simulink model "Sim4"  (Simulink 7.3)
settings: Solver=ode45  StartTime=0.0  StopTime=60  FixedStep=0.01  RelTol=1e-3
InitFcn:
  | r2d=180/pi; d2r=pi/180;
  | om=1.2; zt=0.14; Kp=om^2; Kr=2*zt*om; %frq;
  | [Ad, Bd, Cd, Dd]= later_des;
  | [An, Bn, Cn, Dn]= later_anal;
  | [Ap, Bp, Cp, Dp]= plant;
  | load TVC.mat -ascii
  | 
  | Mass=93215; Sref= 2690; Qbar=745.4; Cyb=-0.0353;
  | Thr=[470000, 470000, 470000, 0.245e7, 0.245e7]';
StopFcn:
  | pl
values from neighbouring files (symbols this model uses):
  Kl3 = INFO.KFI(:,1:7)    [run.m]
  Kp3 = INFO.KFI(:,1:5)    [run.m]
undefined symbols (not defined in the file or in its folder): Ap, Bp, Cp, Cza, Dp, TVC

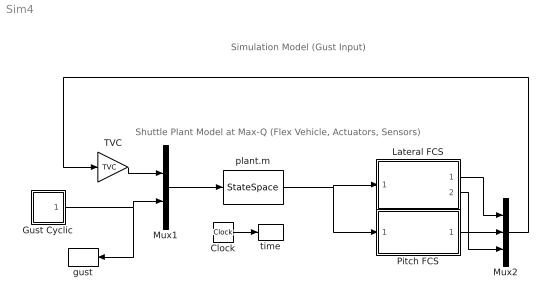
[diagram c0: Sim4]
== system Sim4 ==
  note: Shuttle Plant Model at Max-Q (Flex Vehicle, Actuators, Sensors)
  note: Simulation Model (Gust Input)
  Clock : Clock
  Gust Cyclic : Subsystem
  Lateral FCS : Subsystem
  Mux1 : Mux  Inputs=[10,1]
  Mux2 : Mux  Inputs=3
  Pitch FCS : Subsystem
  TVC : Gain  Gain=TVC  Multiplication=Matrix(K*u)  ParameterDataType=sfix(16)  ParameterScaling=2^0  OutDataType=sfix(16)  OutScaling=2^0
  gust : ToWorkspace  VariableName=gust  SampleTime=-1  SaveFormat=Array
  plant.m : StateSpace  A=Ap  B=Bp  C=Cp  D=Dp
  time : ToWorkspace  VariableName=time  SampleTime=-1  SaveFormat=Array
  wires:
  Mux1/1 -> plant.m/1
  TVC/1 -> Mux1/1
  Clock/1 -> time/1
  plant.m/1 -> Lateral FCS/1(ym), Pitch FCS/1(ym)
  Lateral FCS/1(dP) -> Mux2/1
  Lateral FCS/2(dR) -> Mux2/3
  Mux2/1 -> TVC/1
  Pitch FCS/1(dQ) -> Mux2/2
  Gust Cyclic/1(Gust) -> Mux1/2, gust/1

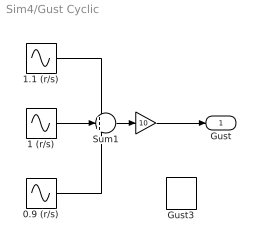
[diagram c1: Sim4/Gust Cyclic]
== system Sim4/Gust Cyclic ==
  " " : Gain  Gain=10  ParameterDataType=sfix(16)  ParameterScaling=2^0  OutDataType=sfix(16)  OutScaling=2^0
  0.9 (r/s) : Sin  Amplitude=1  Bias=0  Frequency=0.9  Phase=0  Samples=10  SampleTime=0
  1 (r/s) : Sin  Amplitude=1  Bias=0  Frequency=1  Phase=0  Samples=10  SampleTime=0
  1.1 (r/s) : Sin  Amplitude=1  Bias=0  Frequency=1.1  Phase=0  Samples=10  SampleTime=0
  Gust3 : DiscretePulseGenerator  PulseType=Time based  Amplitude=36  Period=100  PulseWidth=2  PhaseDelay=0  SampleTime=1
  Sum1 : Sum  Inputs=+++  OutDataType=fixdt(1, 16)  OutScaling=2^0
  Gust : Outport
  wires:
  " "/1 -> Gust/1
  1.1 (r/s)/1 -> Sum1/1
  1 (r/s)/1 -> Sum1/2
  0.9 (r/s)/1 -> Sum1/3
  Sum1/1 -> " "/1

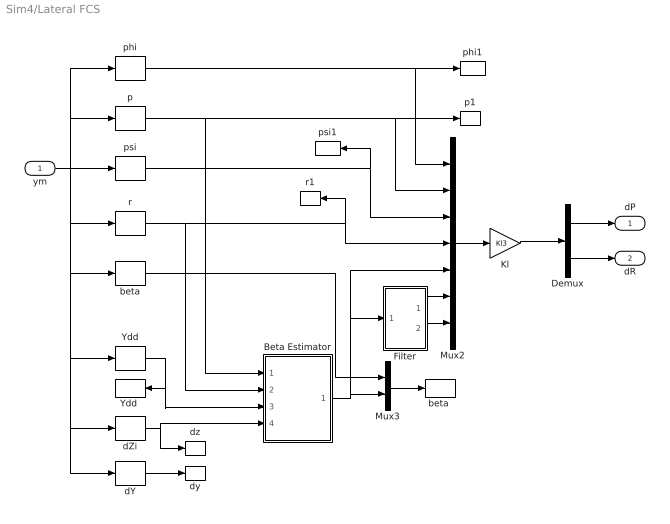
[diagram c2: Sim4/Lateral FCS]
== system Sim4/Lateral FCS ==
  ym : Inport
  Beta Estimator : Subsystem
  Demux : Demux  Outputs=2
  Filter : Subsystem
  Kl : Gain  Gain=Kl3  Multiplication=Matrix(K*u)  ParameterDataType=sfix(16)  ParameterScaling=2^0  OutDataType=sfix(16)  OutScaling=2^0
  Mux2 : Mux  Inputs=7
  Mux3 : Mux  Inputs=2
  Ydd : Selector  InputPortWidth=30  IndexOptions=Index vector (dialog)  Indices=[7]  OutputSizes=1
  "Ydd " : ToWorkspace  VariableName=Ydd  SampleTime=-1  SaveFormat=Array
  beta : Selector  InputPortWidth=30  IndexOptions=Index vector (dialog)  Indices=[10]  OutputSizes=1
  "beta " : ToWorkspace  VariableName=beta  SampleTime=-1  SaveFormat=Array
  dY : Selector  InputPortWidth=30  IndexOptions=Index vector (dialog)  Indices=[21:25]  OutputSizes=1
  dZi : Selector  InputPortWidth=30  IndexOptions=Index vector (dialog)  Indices=[26:30]  OutputSizes=1
  dy : ToWorkspace  VariableName=dy  SampleTime=-1  SaveFormat=Array
  dz : ToWorkspace  VariableName=dz  SampleTime=-1  SaveFormat=Array
  p : Selector  InputPortWidth=30  IndexOptions=Index vector (dialog)  Indices=[4]  OutputSizes=1
  p1 : ToWorkspace  VariableName=p  SampleTime=-1  SaveFormat=Array
  phi : Selector  InputPortWidth=30  IndexOptions=Index vector (dialog)  Indices=[1]  OutputSizes=1
  phi1 : ToWorkspace  VariableName=phi  SampleTime=-1  SaveFormat=Array
  psi : Selector  InputPortWidth=30  IndexOptions=Index vector (dialog)  Indices=[3]  OutputSizes=1
  psi1 : ToWorkspace  VariableName=psi  SampleTime=-1  SaveFormat=Array
  r : Selector  InputPortWidth=30  IndexOptions=Index vector (dialog)  Indices=[6]  OutputSizes=1
  r1 : ToWorkspace  VariableName=r  SampleTime=-1  SaveFormat=Array
  dP : Outport
  dR : Outport  Port=2
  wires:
  Mux2/1 -> Kl/1
  Filter/1(x1) -> Mux2/6
  Filter/2(x2) -> Mux2/7
  phi/1 -> Mux2/1, phi1/1
  p/1 -> Beta Estimator/1(p), Mux2/2, p1/1
  psi/1 -> Mux2/3, psi1/1
  r/1 -> Beta Estimator/2(r), Mux2/4, r1/1
  ym/1 -> p/1, phi/1, psi/1, dY/1, dZi/1, Ydd/1, beta/1, r/1
  Ydd/1 -> Beta Estimator/3(Ydd), "Ydd "/1
  dZi/1 -> Beta Estimator/4(dz), dz/1
  Beta Estimator/1(bethat) -> Mux3/2, Filter/1(bet), Mux2/5
  Mux3/1 -> "beta "/1
  dY/1 -> dy/1
  Kl/1 -> Demux/1
  Demux/2 -> dR/1
  Demux/1 -> dP/1
  beta/1 -> Mux3/1

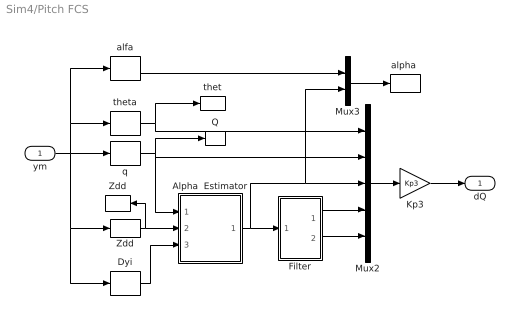
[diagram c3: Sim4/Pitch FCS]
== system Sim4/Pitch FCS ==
  ym : Inport
  " Zdd " : ToWorkspace  VariableName=Zdd  SampleTime=-1  SaveFormat=Array
  Alpha  Estimator : Subsystem
  Dyi : Selector  InputPortWidth=30  IndexOptions=Index vector (dialog)  Indices=[21:25]  OutputSizes=1
  Filter : Subsystem
  Kp3 : Gain  Gain=Kp3  Multiplication=Matrix(K*u)  ParameterDataType=sfix(16)  ParameterScaling=2^0  OutDataType=sfix(16)  OutScaling=2^0
  Mux2 : Mux  Inputs=5
  Mux3 : Mux  Inputs=2
  Q : ToWorkspace  VariableName=q  SampleTime=-1  SaveFormat=Array
  Zdd : Selector  InputPortWidth=30  IndexOptions=Index vector (dialog)  Indices=[8]  OutputSizes=1
  alfa : Selector  InputPortWidth=30  IndexOptions=Index vector (dialog)  Indices=[9]  OutputSizes=1
  "alpha " : ToWorkspace  VariableName=alfa  SampleTime=-1  SaveFormat=Array
  q : Selector  InputPortWidth=30  IndexOptions=Index vector (dialog)  Indices=[5]  OutputSizes=1
  thet : ToWorkspace  VariableName=thet  SampleTime=-1  SaveFormat=Array
  theta : Selector  InputPortWidth=30  IndexOptions=Index vector (dialog)  Indices=[2]  OutputSizes=1
  dQ : Outport
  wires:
  Kp3/1 -> dQ/1
  Dyi/1 -> Alpha  Estimator/3(delta)
  Zdd/1 -> Alpha  Estimator/2(Zdd), " Zdd "/1
  Alpha  Estimator/1(alphat) -> Filter/1(alfa), Mux2/3, Mux3/2
  ym/1 -> q/1, Zdd/1, Dyi/1, theta/1, alfa/1
  q/1 -> Alpha  Estimator/1(q), Mux2/2, Q/1
  theta/1 -> Mux2/1, thet/1
  Filter/2(x2) -> Mux2/5
  Filter/1(x1) -> Mux2/4
  Mux2/1 -> Kp3/1
  Mux3/1 -> "alpha "/1
  alfa/1 -> Mux3/1

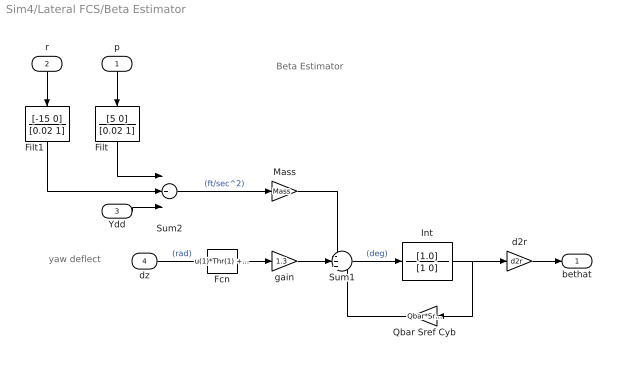
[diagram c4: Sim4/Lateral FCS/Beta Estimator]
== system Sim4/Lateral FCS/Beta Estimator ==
  note: Beta Estimator
  note: yaw deflect
  p : Inport
  r : Inport  Port=2
  Ydd : Inport  Port=3
  dz : Inport  Port=4  OutDataType=sfix(16)  OutScaling=2^0
  Fcn : Fcn  Expr=u(1)*Thr(1) +u(2)*Thr(2) +u(3)*Thr(3) +u(4)*Thr(4) +u(5)*Thr(5)
  Filt : TransferFcn  Numerator=[5 0]  Denominator=[0.02 1]
  Filt1 : TransferFcn  Numerator=[-15 0]  Denominator=[0.02 1]
  Int : TransferFcn  Numerator=[1.0]  Denominator=[1 0]
  Mass : Gain  Gain=Mass  ParameterDataType=sfix(16)  ParameterScaling=2^0  OutDataType=sfix(16)  OutScaling=2^0
  Qbar Sref Cyb : Gain  Gain=Qbar*Sref*Cyb  ParameterDataType=sfix(16)  ParameterScaling=2^0  OutDataType=sfix(16)  OutScaling=2^0
  Sum1 : Sum  Inputs=-++  OutDataType=sfix(16)  OutScaling=2^0
  Sum2 : Sum  Inputs=+++  OutDataType=sfix(16)  OutScaling=2^0
  d2r : Gain  Gain=d2r  ParameterDataType=sfix(16)  ParameterScaling=2^0  OutDataType=sfix(16)  OutScaling=2^0
  gain : Gain  Gain=1.3  ParameterDataType=sfix(16)  ParameterScaling=2^0  OutDataType=sfix(16)  OutScaling=2^0
  bethat : Outport  OutDataType=sfix(16)  OutScaling=2^0
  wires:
  Filt1/1 -> Sum2/2
  Sum1/1 -> Int/1  "(deg)"
  Qbar Sref Cyb/1 -> Sum1/3
  dz/1 -> Fcn/1  "(rad)"
  Sum2/1 -> Mass/1  "(ft/sec^2)"
  Mass/1 -> Sum1/1
  d2r/1 -> bethat/1
  Int/1 -> d2r/1, Qbar Sref Cyb/1
  Fcn/1 -> gain/1
  gain/1 -> Sum1/2
  Ydd/1 -> Sum2/3
  r/1 -> Filt1/1
  p/1 -> Filt/1
  Filt/1 -> Sum2/1

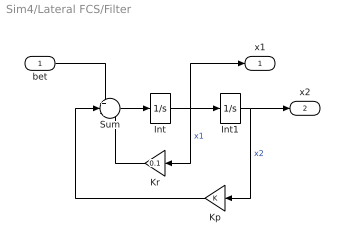
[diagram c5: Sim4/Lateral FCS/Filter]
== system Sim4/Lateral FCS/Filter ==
  bet : Inport  OutDataType=sfix(16)  OutScaling=2^0
  Int : Integrator
  Int1 : Integrator
  Kp : Gain  ParameterDataType=sfix(16)  ParameterScaling=2^0  OutDataType=sfix(16)  OutScaling=2^0
  Kr : Gain  Gain=0.1  ParameterDataType=sfix(16)  ParameterScaling=2^0  OutDataType=sfix(16)  OutScaling=2^0
  Sum : Sum  Inputs=+--  OutDataType=sfix(16)  OutScaling=2^0
  x1 : Outport  OutDataType=sfix(16)  OutScaling=2^0
  x2 : Outport  Port=2  OutDataType=sfix(16)  OutScaling=2^0
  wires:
  Int/1 -> Int1/1, Kr/1, x1/1  "x1"
  Sum/1 -> Int/1
  Int1/1 -> Kp/1, x2/1  "x2"
  Kr/1 -> Sum/3
  Kp/1 -> Sum/2
  bet/1 -> Sum/1

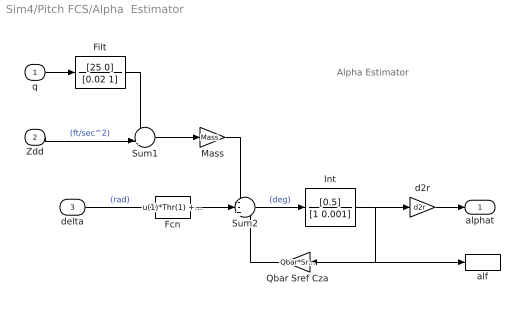
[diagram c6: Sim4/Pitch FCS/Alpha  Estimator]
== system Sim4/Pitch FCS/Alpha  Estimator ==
  note: Alpha Estimator
  q : Inport  OutDataType=sfix(16)  OutScaling=2^0
  Zdd : Inport  Port=2  OutDataType=sfix(16)  OutScaling=2^0
  delta : Inport  Port=3  OutDataType=sfix(16)  OutScaling=2^0
  Fcn : Fcn  Expr=u(1)*Thr(1) +u(2)*Thr(2) +u(3)*Thr(3) +u(4)*Thr(4) +u(5)*Thr(5)
  Filt : TransferFcn  Numerator=[25 0]  Denominator=[0.02 1]
  Int : TransferFcn  Numerator=[0.5]  Denominator=[1 0.001]
  Mass : Gain  Gain=Mass  ParameterDataType=sfix(16)  ParameterScaling=2^0  OutDataType=sfix(16)  OutScaling=2^0
  Qbar Sref Cza : Gain  Gain=Qbar*Sref*Cza  ParameterDataType=sfix(16)  ParameterScaling=2^0  OutDataType=sfix(16)  OutScaling=2^0
  Sum1 : Sum  Inputs=++|  OutDataType=sfix(16)  OutScaling=2^0
  Sum2 : Sum  Inputs=--+  OutDataType=sfix(16)  OutScaling=2^0
  alf : ToWorkspace  VariableName=alphat  SampleTime=-1  SaveFormat=Array
  d2r : Gain  Gain=d2r  ParameterDataType=sfix(16)  ParameterScaling=2^0  OutDataType=sfix(16)  OutScaling=2^0
  alphat : Outport  OutDataType=sfix(16)  OutScaling=2^0
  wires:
  Fcn/1 -> Sum2/2
  Filt/1 -> Sum1/1
  Sum1/1 -> Mass/1
  Zdd/1 -> Sum1/2  "(ft/sec^2)"
  q/1 -> Filt/1
  Sum2/1 -> Int/1  "(deg)"
  Qbar Sref Cza/1 -> Sum2/3
  delta/1 -> Fcn/1  "(rad)"
  Mass/1 -> Sum2/1
  d2r/1 -> alphat/1
  Int/1 -> d2r/1, Qbar Sref Cza/1, alf/1

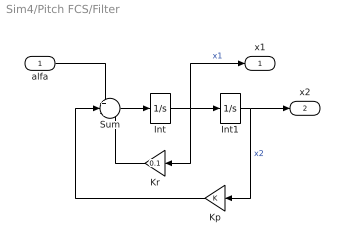
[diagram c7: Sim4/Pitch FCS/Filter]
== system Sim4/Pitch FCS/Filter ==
  alfa : Inport  OutDataType=sfix(16)  OutScaling=2^0
  Int : Integrator
  Int1 : Integrator
  Kp : Gain  ParameterDataType=sfix(16)  ParameterScaling=2^0  OutDataType=sfix(16)  OutScaling=2^0
  Kr : Gain  Gain=0.1  ParameterDataType=sfix(16)  ParameterScaling=2^0  OutDataType=sfix(16)  OutScaling=2^0
  Sum : Sum  Inputs=+--  OutDataType=sfix(16)  OutScaling=2^0
  x1 : Outport  OutDataType=sfix(16)  OutScaling=2^0
  x2 : Outport  Port=2  OutDataType=sfix(16)  OutScaling=2^0
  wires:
  alfa/1 -> Sum/1
  Kp/1 -> Sum/2
  Kr/1 -> Sum/3
  Int1/1 -> x2/1, Kp/1  "x2"
  Sum/1 -> Int/1
  Int/1 -> x1/1, Kr/1, Int1/1  "x1"
